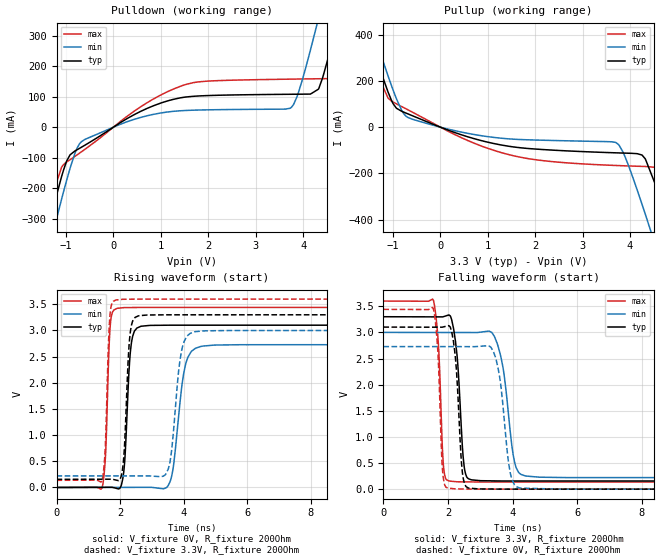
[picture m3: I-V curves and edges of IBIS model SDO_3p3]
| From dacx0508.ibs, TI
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|   Model
[Model]   SDO_3p3
Model_type   Output
Polarity   Non-Inverting
Vmeas = 1.65
Vref = 0
Cref = 1pF
Rref = 100000
|   typ   min   max
C_comp   2.1759pF   1.7605pF   2.60399pF
| Where nom  PVT is Nominal Process, 3.3V, 27C
|   Fast PVT is Strong Process,  3.6V, -40C
|   Slow PVT is Weak Process,   3.0V, 125C
[Voltage Range]   3.3   3   3.6
|Junction Temperature
[Temperature Range]   27   125   -40
[Pullup Reference]   3.3   3   3.6
[Pulldown Reference]   -0   -0   -0
[Power Clamp Reference]   3.3   3   3.6
[GND Clamp Reference]   0   0   0
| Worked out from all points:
|   slope of the pulldown table from 0 to 0.495 V, typ, clamps not added: 10.9 ohm
|   slope of the pullup table from 0 to 0.495 V, typ, clamps not added: 13.6 ohm
|   falling waveform, V_fixture 3.3V, R_fixture 200Ohm: 20-80 % time 188ps typ, 322ps min, 136ps max; typ from 3.3 V to 0.156 V
|   rising waveform, V_fixture 0V, R_fixture 200Ohm: 20-80 % time 151ps typ, 298ps min, 110ps max; typ from 0 V to 3.1 V
|   rising waveform, V_fixture 3.3V, R_fixture 200Ohm: 20-80 % time 140ps typ, 254ps min, 107ps max; typ from 0.156 V to 3.3 V
|   falling waveform, V_fixture 0V, R_fixture 200Ohm: 20-80 % time 170ps typ, 278ps min, 128ps max; typ from 3.1 V to 0 V
[Pulldown]
|   Voltage   I(typ)   I(min)   I(max)
-3.3V     -1.58A     -1.658A    -1.532A
-1.468V   -387.5mA   -467.7mA   -337.1mA
-1.251V   -252.8mA   -331.6mA   -205.3mA
-983.4mV  -110.3mA   -172.6mA   -114.2mA
-716.1mV  -69.62mA   -54.88mA   -85.51mA
264mV     25.92mA    16.41mA    32.71mA
1.68V     101.1mA    55.63mA    145.8mA
3.729V    107.8mA    62.53mA    157.5mA
4.323V    124.7mA    356.3mA    158.8mA
4.709V    335.7mA    599.9mA    161.8mA
5.224V    663.4mA    932.2mA    424.7mA
6.6V      1.564A     1.833A     1.322A
[Pullup]
|   Voltage   I(typ)   I(min)   I(max)
-3.3V     1.564A     1.636A     1.52A
-1.894V   643.6mA    718.6mA    597mA
-1.449V   358.9mA    434.2mA    312.5mA
-993.3mV  100.8mA    159.1mA    108.3mA
-577.5mV  48.31mA    33.46mA    63.52mA
1.403V    -81.3mA    -50mA      -116.6mA
3.709V    -111.1mA   -67.46mA   -165.8mA
4.254V    -120.6mA   -334.3mA   -169.7mA
4.561V    -261.3mA   -526.6mA   -174.3mA
4.877V    -457.5mA   -729.4mA   -230.3mA
5.234V    -686.2mA   -960.2mA   -444.3mA
6.6V      -1.581A    -1.855A    -1.335A
[Ramp]
R_load = 200
|   typ   min   max
dV/dt_r   1.86109/1.50994e-10   1.63721/2.96285e-10   2.06456/1.10255e-10
dV/dt_f   1.88659/1.86485e-10   1.66786/3.21439e-10   2.07818/1.35913e-10
[Falling Waveform]
V_fixture = 3.3V
V_fixture_min = 3V
V_fixture_max = 3.6V
R_fixture = 200Ohm
C_fixture = 0F
|   Time   V(typ)   V(min)   V(max)
0s        3.3V       3V         3.6V
1.548ns   3.297V     2.999V     3.614V
1.704ns   3.297V     2.999V     2.752V
1.856ns   3.301V     2.998V     463mV
2.026ns   3.334V     2.998V     158.5mV
2.497ns   440.9mV    2.998V     139.8mV
2.703ns   182.4mV    2.998V     138.6mV
3.517ns   157.9mV    2.795V     137mV
4.372ns   156.6mV    256.7mV    137mV
20ns      155.7mV    220.2mV    136.3mV
[Rising Waveform]
V_fixture = 0V
V_fixture_min = 0V
V_fixture_max = 0V
R_fixture = 200Ohm
C_fixture = 0F
|   Time   V(typ)   V(min)   V(max)
0s        15.95uV    23.35uV    11.56uV
1.434ns   2.457mV    1.108mV    -7.236mV
1.696ns   2.903mV    1.305mV    3.122V
1.898ns   -19.38mV   1.458mV    3.421V
2.358ns   2.758V     1.806mV    3.438V
2.649ns   3.078V     2.026mV    3.44V
3.571ns   3.101V     104.2mV    3.44V
4.054ns   3.101V     2.324V     3.44V
4.53ns    3.101V     2.692V     3.44V
20ns      3.102V     2.729V     3.441V
[Rising Waveform]
V_fixture = 3.3V
V_fixture_min = 3V
V_fixture_max = 3.6V
R_fixture = 200Ohm
C_fixture = 0F
|   Time   V(typ)   V(min)   V(max)
0s        155.7mV    220.2mV    136.3mV
1.434ns   157.5mV    220.6mV    132.8mV
1.68ns    157.9mV    220.6mV    3.266V
1.863ns   142.7mV    220.7mV    3.581V
2.326ns   2.979V     220.8mV    3.597V
2.575ns   3.278V     220.9mV    3.599V
3.517ns   3.299V     349.6mV    3.599V
3.937ns   3.299V     2.606V     3.599V
4.342ns   3.299V     2.973V     3.599V
20ns      3.3V       3V         3.6V
[Falling Waveform]
|Gnd
V_fixture = 0V
V_fixture_min = 0V
V_fixture_max = 0V
R_fixture = 200Ohm
C_fixture = 0F
|   Time   V(typ)   V(min)   V(max)
0s        3.102V     2.729V     3.441V
1.541ns   3.1V       2.728V     3.462V
1.688ns   3.1V       2.728V     2.598V
1.83ns    3.101V     2.728V     361.6mV
1.988ns   3.125V     2.728V     21.5mV
2.625ns   22.97mV    2.728V     2.213mV
3.408ns   2.316mV    2.628V     708.6uV
3.921ns   756.5uV    324.4mV    687.1uV
4.211ns   743.1uV    23.03mV    674.9uV
20ns      15.84uV    23.58uV    11.56uV
